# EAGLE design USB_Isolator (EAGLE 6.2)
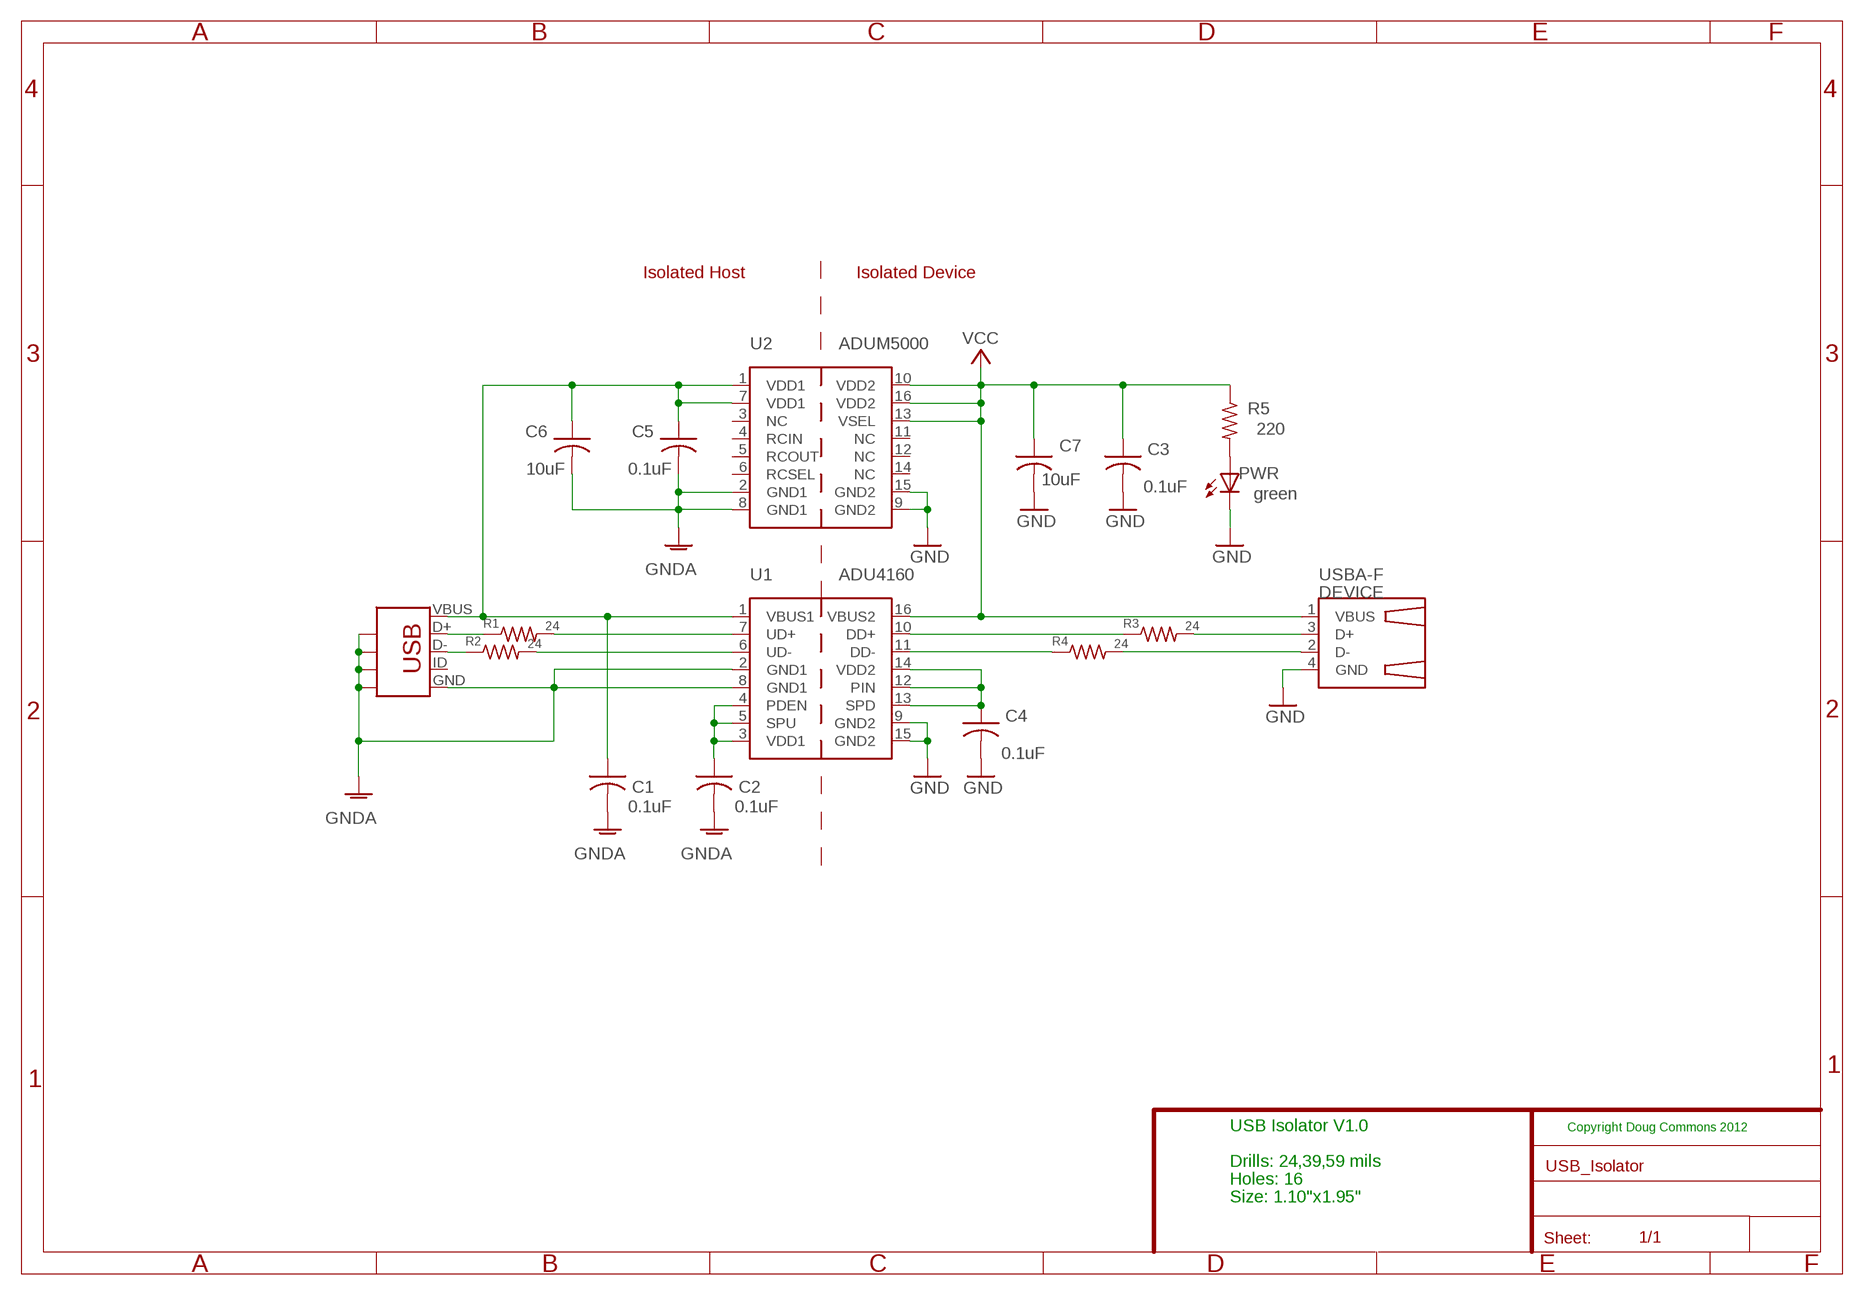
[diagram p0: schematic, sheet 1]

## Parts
C1  0.1uF  C-USC0603  [C0603]
C2  0.1uF  C-USC0603  [C0603]
C3  0.1uF  C-USC0603  [C0603]
C4  0.1uF  C-USC0603  [C0603]
C5  0.1uF  C-USC0603  [C0603]
C6  10uF  C-USC0805  [C0805]
C7  10uF  C-USC0805  [C0805]
DEVICE  USBA-F  [USBA-F]
HOST  USB  [USB-MB-S]
PWR  green  LEDCHIPLED_1206  [CHIPLED_1206]
R1  24  R-US_R0603  [R0603]
R2  24  R-US_R0603  [R0603]
R3  24  R-US_R0603  [R0603]
R4  24  R-US_R0603  [R0603]
R5  220  R-US_R0603  [R0603]
U1  ADU4160  [SO16L]
U2  ADUM5000  [SO16L]

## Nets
DD+: R3.1 U1.10(DD+)
DD-: R4.1 U1.11(DD-)
GND [gnd]: C3.2 C4.2 C7.2 DEVICE.4(GND) PWR.C U1.9(GND2) U1.15(GND2) U2.9(GND2) U2.15(GND2)
GNDA [gnda]: C1.2 C2.2 C5.2 C6.2 HOST.GND HOST.GND@1(GND1) HOST.GND@2(GND2) HOST.GND@3(GND3) HOST.GND@4(GND4) U1.2(GND1) U1.8(GND1) U2.2(GND1) U2.8(GND1)
N$1: DEVICE.3(D+) R3.2
N$2: DEVICE.2(D-) R4.2
N$3: PWR.A R5.2
N$4: C4.1 U1.12(PIN) U1.13(SPD) U1.14(VDD2)
N$41: C2.1 U1.3(VDD1) U1.4(PDEN) U1.5(SPU)
UD+: R1.2 U1.7(UD+)
UD-: R2.2 U1.6(UD-)
UUD+: HOST.D+ R1.1
UUD-: HOST.D- R2.1
VBUS [vbus]: C1.1 C5.1 C6.1 HOST.VBUS U1.1(VBUS1) U2.1(VDD1) U2.7(VDD1)
VCC [vcc]: C3.1 C7.1 DEVICE.1(VBUS) R5.1 U1.16(VBUS2) U2.10(VDD2) U2.13(VSEL) U2.16(VDD2)
Unconnected: HOST.ID(UID) U2.3(NC) U2.4(RCIN) U2.5(RCOUT) U2.6(RCSEL) U2.11(NC) U2.12(NC) U2.14(NC)

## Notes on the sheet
- Isolated Host | Isolated Device
- USB Isolator V1.0 | Copyright Doug Commons 2012
- Drills: 24,39,59 mils
- Holes: 16
- Size: 1.10"x1.95"

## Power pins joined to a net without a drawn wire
GND: DEVICE.5(GND) DEVICE.6(GND) DEVICE.7(GND) DEVICE.8(GND)

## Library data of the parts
C1-C7 = 1_Dougs_custom:C-US: CAPACITOR, American symbol
DEVICE = 1_Dougs_custom:USBA-F
HOST = 1_Dougs_custom:USB: USB Connectors
PWR = led:LED: LED
R1-R5 = 1_Dougs_custom:R-US_: RESISTOR, American symbol
U1 = 1_scope:ADU4160
U2 = 1_scope:ADUM5000

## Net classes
0 default: width 0.254 mm, drill 0.61 mm
2 vcc: width 0.508 mm, drill 0.61 mm
3 gnda: width 0.508 mm, drill 0.61 mm
4 vbus: width 0.508 mm, drill 0.61 mm
5 gnd: width 0.508 mm, drill 0.61 mm

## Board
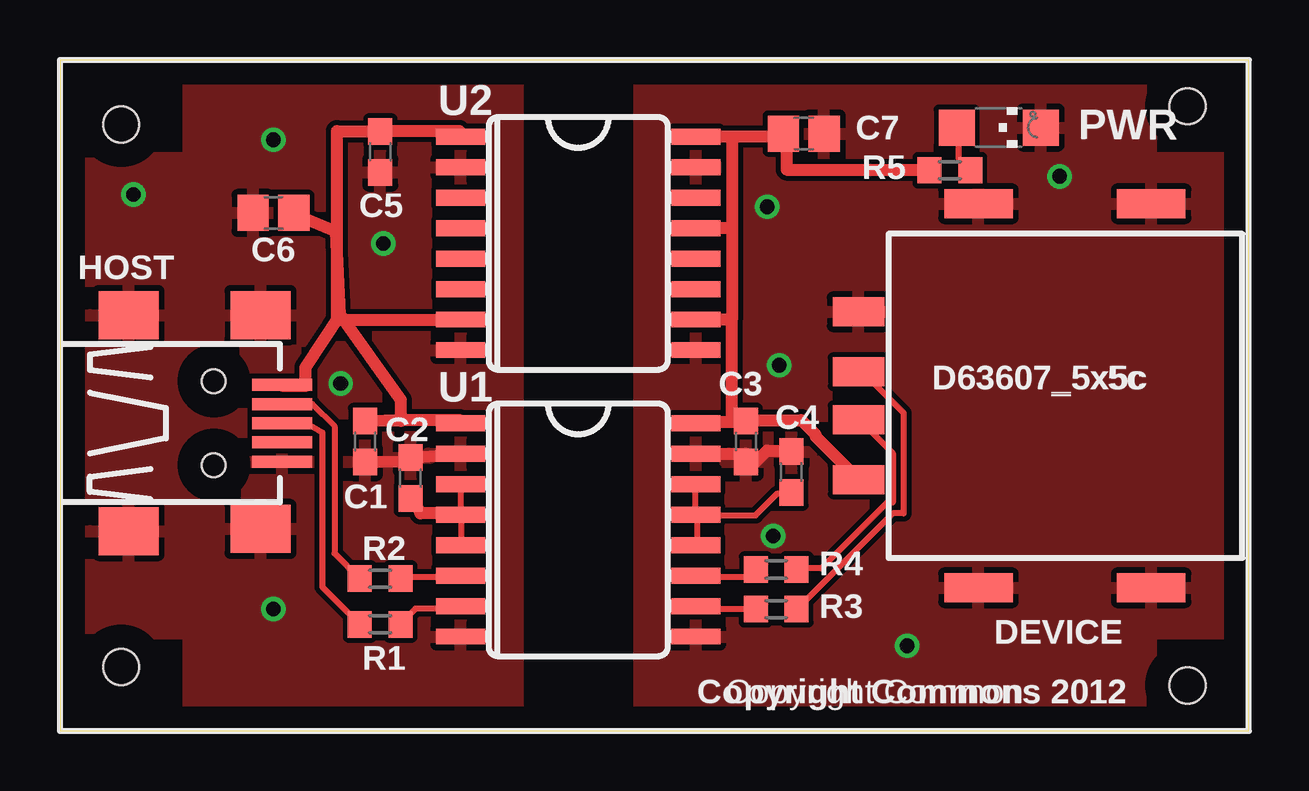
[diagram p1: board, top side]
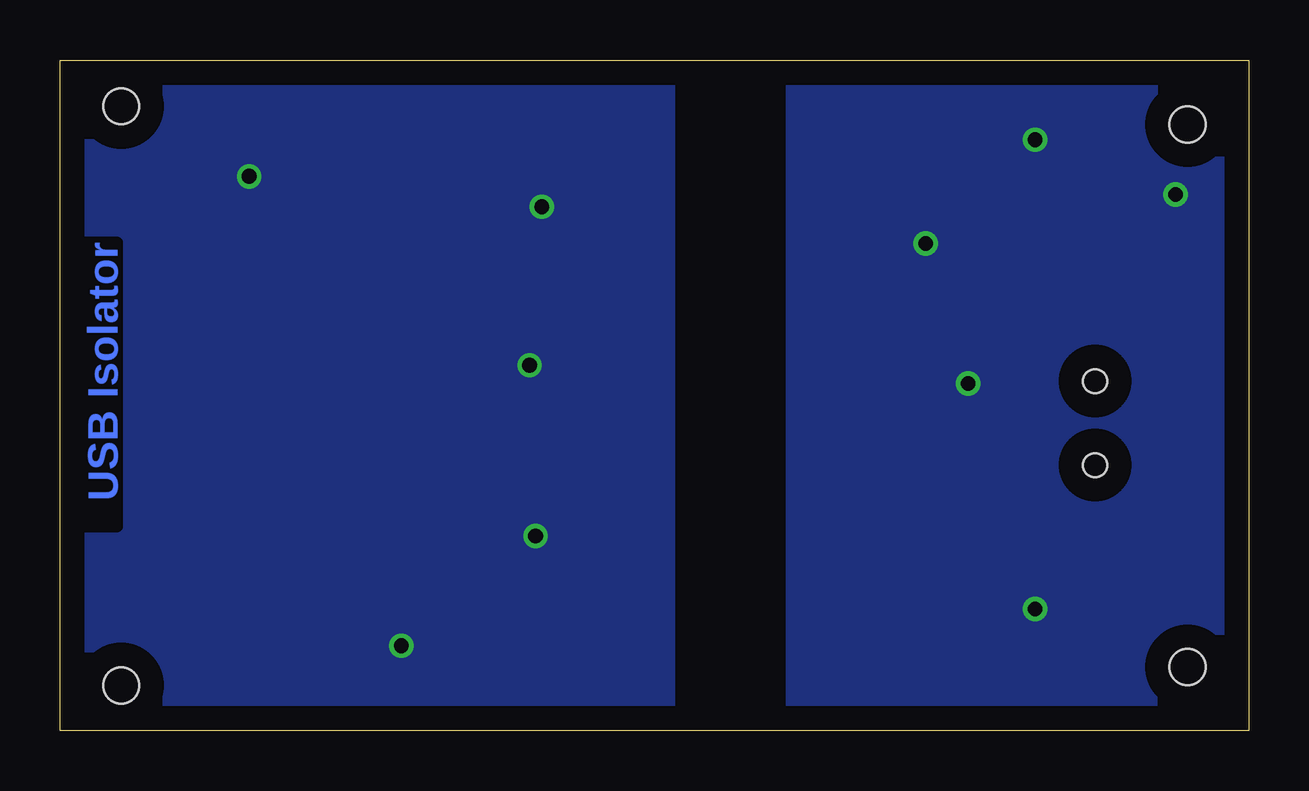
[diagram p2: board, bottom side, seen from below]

Size 49.56 x 27.96 mm. Coordinates in mm from the lower left corner, seen from the top.
Outline: 0,0 49.56,0 49.56,27.96 0,27.96 0,0
Copper layers (1*16): Top 0.035mm / dielectric 1.5mm / Bottom 0.035mm
Design rules: minimum track width 8mil, minimum drill 20mil, track to track 8mil, track to pad 8mil, pad to pad 8mil, via to via 8mil, smd to smd 8mil, copper to edge 40mil, drill to drill 10mil, minimum pad ring 10mil, minimum via ring 8mil, stop-mask expansion 0mil, vias tented up to drill 0mil, thermal gap 10mil
Holes 1.5 mm at 2.55,25.27 2.55,2.66 47,1.9 47,26.03
tRestrict: area 0,24.1 to 5.1,27.9; area 0,0 to 5.1,3.8; area 45.7,24.1 to 50.8,27.9; area 45.7,0 to 50.8,3.8

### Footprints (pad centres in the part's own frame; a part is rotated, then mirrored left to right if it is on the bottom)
C0603 = smd 1.1 x 1: 1 -0.85,0; 2 0.85,0
C0805 = smd 1.3 x 1.5: 1 -0.85,0; 2 0.85,0
USBA-F = smd 1.2 x 2.15: 1 3.5,0; 2 1,0; 3 -1,0; 4 -3.5,0 | smd 1.2 x 2.85: 5 -8,5; 6 -8,12.2; 7 8,12.2; 8 8,5
USB-MB-S = smd 0.5 x 2.5: D+ 0,-9.25; D- 0.8,-9.25; GND -1.6,-9.25; ID -0.8,-9.25; VBUS 1.6,-9.25 | smd 2 x 2.5: GND@1 4.5,-2.842; GND@2 4.5,-8.342; GND@3 -4.5,-2.842; GND@4 -4.4,-8.342 | hole 0.991: -1.75,-6.4; 1.75,-6.4
CHIPLED_1206 = smd 1.5 x 1.5: A 0,-1.75; C 0,1.75
R0603 = smd 1 x 1.1: 1 -0.85,0; 2 0.85,0
SO16L = smd 0.66 x 2.032: 1 -4.445,-4.902; 2 -3.175,-4.902; 3 -1.905,-4.902; 4 -0.635,-4.902; 5 0.635,-4.902; 6 1.905,-4.902; 7 3.175,-4.902; 8 4.445,-4.902; 9 4.445,4.902; 10 3.175,4.902; 11 1.905,4.902; 12 0.635,4.902; 13 -0.635,4.902; 14 -1.905,4.902; 15 -3.175,4.902; 16 -4.445,4.902

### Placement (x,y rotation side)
C1  12.71,12.06 270 top
C2  14.62,10.54 90 top
C3  28.59,12.06 270 top
C4  30.49,10.79 90 top
C5  13.35,24.12 270 top
C6  8.9,21.59 180 top
C7  31,24.89 0 top
DEVICE  33.29,13.96 270 top
HOST  0.01,12.82 90 top
PWR  39.13,25.14 270 top
R1  13.35,4.44 0 top
R2  13.35,6.34 0 top
R3  29.86,5.08 0 top
R4  29.86,6.73 0 top
R5  37.1,23.36 0 top
U1  21.6,8.38 270 top
U2  21.6,20.32 270 top

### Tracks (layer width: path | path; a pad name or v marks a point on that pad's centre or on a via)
DD+
  Top 0.254: R3.1 28.99,5.1 26.56,5.1 26.56,5.18 U1.10
DD-
  Top 0.254: R4.1 28.99,6.42 26.56,6.42 26.56,6.47 U1.11
GND  (via drill 0.61)
  Top 0.508: 28.61,11.2 C3.2 28.59,11.55 U1.15 | 28.61,11.2 C3.2 | 28.61,11.2 28.99,11.2 29.48,11.68 30.45,11.68 C4.2
  other vias: 29.98,15.23 29.73,8.12 41.67,23.11 35.32,3.55 29.48,21.84
  pour Top: 49.54,27.94 24.14,27.94 24.14,-0.01 49.54,-0.01
  pour Bottom: 24.14,27.94 49.54,27.94 49.54,-0.01 24.14,-0.01
GNDA  (via drill 0.61)
  Top 0.508: 14.26,11.2 C1.2 | 14.26,11.2 14.24,11.2 | 14.26,11.2 14.43,11.2 C2.2 U1.2
  other vias: 3.06,22.35 11.7,14.47 8.9,5.08 13.47,20.32 8.9,24.63
  pour Top: 0.01,27.94 19.06,27.94 19.06,-0.01 0.01,-0.01
  pour Bottom: 0.01,27.94 19.06,27.94 19.06,-0.01 0.01,-0.01
N$1
  Top 0.254: R3.2 30.75,5.1 34.71,9.06 35.17,9.06 35.17,13.25 33.49,14.93 33.34,14.93 DEVICE.3
N$2
  Top 0.254: R4.2 30.75,6.78 31.74,6.78 34.48,9.52 34.71,9.52 34.71,11.58 33.34,12.95 DEVICE.2
N$3
  Top 0.254: R5.2 37.91,23.39 37.45,23.85 37.45,25.14 PWR.A
N$4
  Top 0.254: C4.1 30.44,9.9 29.91,9.9 28.99,8.99 26.56,8.99 U1.13 | U1.12 26.56,7.77 26.56,8.91 U1.13 | U1.14 26.48,10.28 26.48,9.14 U1.13
N$41
  Top 0.254: 14.69,9.65 14.36,9.65 C2.1 | 16.65,9.06 U1.4 | U1.5 16.73,7.77 16.73,8.91 U1.4 | U1.3 16.73,10.28 16.73,9.14 U1.4
  Top 0.508: 14.69,9.65 15.02,9.06 16.65,9.06
UD+
  Top 0.254: R1.2 14.21,4.49 14.82,5.1 16.65,5.1 16.65,5.18 U1.7
UD-
  Top 0.254: R2.2 14.21,6.4 16.65,6.4 16.65,6.47 U1.6
UUD+
  Top 0.254: HOST.D+ 10.3,12.82 10.93,12.44 10.93,6 R1.1
UUD-
  Top 0.254: HOST.D- 10.52,13.62 11.44,12.69 11.44,7.4 R2.1
VBUS
  Top 0.508: U2.1 16.65,24.76 16.65,24.99 13.37,24.99 C5.1 13.14,24.99 11.54,24.99 11.54,17.14 11.67,17.14 | U1.1 16.65,12.87 16.65,12.95 14.29,12.95 C1.1 14.21,12.92 14.21,13.79 11.67,17.34 | 11.67,17.34 11.52,20.8 | 11.52,20.8 9.77,21.53 C6.1 | 11.67,17.14 U2.7 | 11.67,17.14 11.52,20.8 | 11.67,17.34 10.22,15.13 10.22,14.37 9.31,14.37 HOST.VBUS
VCC
  Top 0.508: 28,24.76 29.91,24.76 29.91,24.84 C7.1 30.29,24.68 30.29,23.39 36.23,23.39 R5.1 | 28,24.76 U2.16 | 28,12.87 26.56,12.87 U1.16 | 28,12.87 28.54,12.87 C3.1 28.84,12.95 30.9,12.95 31.51,12.34 31.51,12.26 33.26,10.51 DEVICE.1 | 28,17.14 U2.10 | 28,12.87 28,17.14 | 28,20.95 U2.13 | 28,24.76 28,20.95 | 28,20.95 28,17.14

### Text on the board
Bottom: USB Isolator
tPlace: D63607_5x5c | Copyright Commons 2012
_tplace: U2 | C7 | PWR | R5 | C6 | C5 | HOST | U1 | C3 | C4 | D63607_5x5c | C2 | C1 | R2 | R4 | R3 | DEVICE | R1 | Copyright Commons 2012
